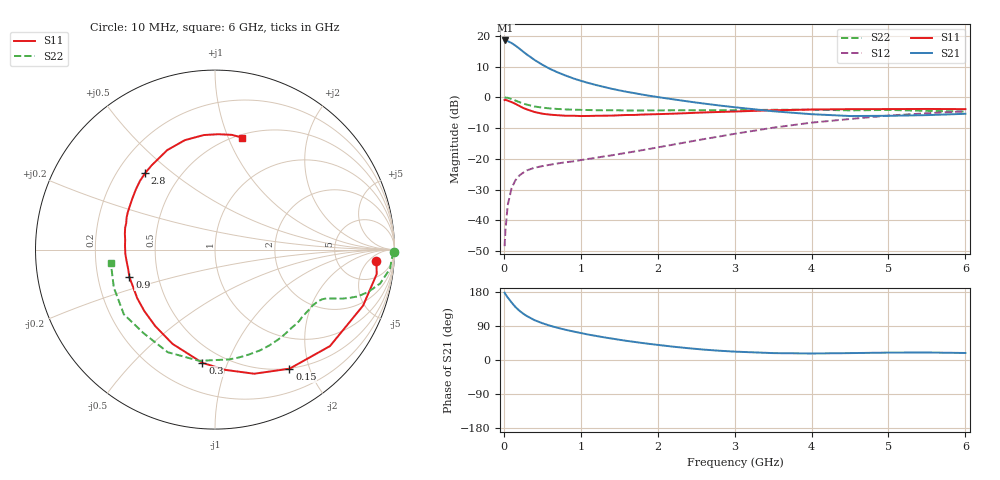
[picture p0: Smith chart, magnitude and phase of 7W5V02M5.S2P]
! Infineon Technologies  Discrete & RF Semiconductors
! BFS17W
! Si NPN RF Bipolar Junction Transistor in SOT323
! VCE = 5 V  IC = 2.5 mA
! Common Emitter S-Parameters:  August  1999
# GHz  S  MA  R  50
!  f  S11  S21  S12  S22
! GHz  MAG  ANG  MAG  ANG  MAG  ANG  MAG  ANG
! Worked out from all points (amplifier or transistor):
!   36 points, 10 MHz to 6 GHz, reference 50 ohm
!   highest |S21| = 18.5 dB at 20 MHz (marker M1)
!   |S21| within 3 dB of that: start of sweep to 219.4 MHz
!   unconditionally stable (mu >= 1): 774.8 MHz to 2.917 GHz; 4.234 GHz to end of sweep
!   at 250 MHz: K = 0.40, MSG = 19.7 dB, |S12| = -24.5 dB
!   at 1.4 GHz: K = 1.27, MAG = 7.7 dB, |S12| = -18.9 dB
!   at 6 GHz: K = 1.08, MAG = -2.1 dB, |S12| = -4.6 dB
!   S11 on the Smith chart (normalised r, x): 10 MHz: 13, -9; 150 MHz: 0.49, -1.70; 300 MHz: 0.39, -0.82; 900 MHz: 0.34, -0.14; 2.8 GHz: 0.32, +0.40; 6 GHz: 0.53, +1.12
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0.01  0.9018 -4.1  8.365 177.6  0.0038 85.3  0.9986 -0.8
0.02  0.9112 -8.6  8.39 174.0  0.0066 89.9  0.9878 -2.5
0.05  0.8821 -20.7  8.179 165.2  0.0175 80.3  0.9806 -6.3
0.1  0.8363 -40.0  7.619 152.0  0.0331 69.0  0.9392 -11.6
0.15  0.7826 -58.0  6.932 140.0  0.0446 60.7  0.8853 -15.5
0.2  0.7251 -72.5  6.216 130.4  0.0533 55.5  0.8359 -18.2
0.25  0.6727 -85.1  5.527 122.5  0.0593 50.5  0.7923 -19.9
0.3  0.6349 -96.3  4.956 115.8  0.0649 47.8  0.7588 -21.1
0.4  0.5763 -114.2  4.039 105.1  0.0717 44.5  0.7087 -22.6
0.5  0.541 -127.9  3.384 97.1  0.076 43.0  0.6789 -23.6
0.6  0.5218 -139.0  2.896 90.5  0.0801 43.3  0.659 -24.8
0.7  0.511 -148.0  2.541 84.9  0.084 44.1  0.6457 -26.2
0.9  0.5012 -162.1  2.035 75.4  0.0907 47.1  0.6275 -29.5
1.1  0.4972 -173.2  1.707 67.0  0.0997 50.0  0.6202 -33.4
1.3  0.5019 177.4  1.474 59.9  0.1092 53.6  0.6138 -37.9
1.6  0.5154 166.2  1.225 50.4  0.1253 58.2  0.6107 -44.8
2.2  0.5413 148.3  0.927 35.2  0.1699 65.2  0.614 -60.5
2.8  0.577 132.4  0.736 24.5  0.2305 66.9  0.6157 -77.5
3.5  0.6148 115.7  0.593 18.2  0.3204 63.8  0.626 -98.1
4.5  0.6413 95.6  0.496 18.2  0.4437 52.0  0.6125 -130.3
5.5  0.6461 81.6  0.513 19.8  0.5501 38.9  0.6022 -159.4
6  0.6419 76.4  0.539 18.5  0.591 32.5  0.5851 -172.4
